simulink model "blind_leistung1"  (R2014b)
settings: Solver=ode8  StartTime=0.0  StopTime=5  FixedStep=1e-5  RelTol=1e-3
undefined symbols (not defined in the file or in its folder): fdesignblkfcn, fir1, gcbh
libraries: dsparch4 x2, dspsigops x1

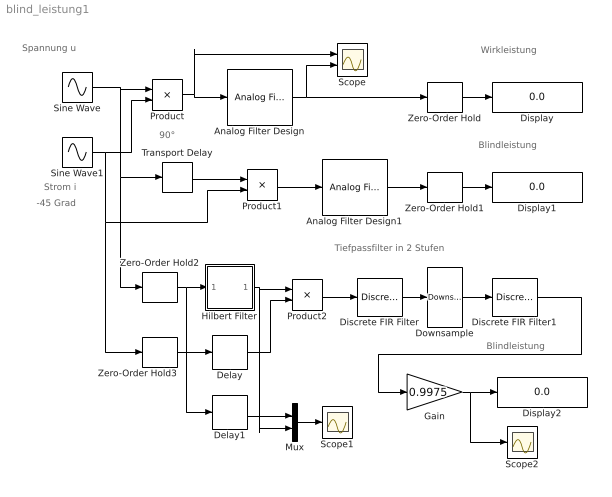
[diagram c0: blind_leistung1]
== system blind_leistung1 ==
  note: Tiefpassfilter in 2 Stufen
  note: Blindleistung
  note: Blindleistung
  note: Wirkleistung
  note: 90°
  note: -45 Grad
  note: Strom i
  note: Spannung u
  Analog Filter Design : dsparch4/Analog Filter Design  method=Butterworth  filttype=Lowpass  N=8  Wlo=2*pi*10  Whi=80  Rp=2  Rs=40
  Analog Filter Design1 : dsparch4/Analog Filter Design  method=Butterworth  filttype=Lowpass  N=8  Wlo=2*pi*10  Whi=80  Rp=2  Rs=40
  Delay : Delay  DelayLength=32
  Delay1 : Delay  DelayLength=32
  Discrete FIR Filter : DiscreteFir  Coefficients=fir1(128, 50*2/1000)
  Discrete FIR Filter1 : DiscreteFir  Coefficients=fir1(128, 10*2/200)
  Display : Display
  Display1 : Display
  Display2 : Display
  Downsample : dspsigops/Downsample  N=5  phase=0  RateOptions=Allow multirate processing  smode=Allow multirate  fmode=Maintain input frame size  ic=0
  Gain : Gain  Gain=0.9975
  Hilbert Filter : Subsystem  DialogController=fdesignblkfcn  InitFcn=fdesignblkfcn(gcbh, {'InitFcn'});
  Mux : Mux  Inputs=2
  Product : Product
  Product1 : Product
  Product2 : Product
  Scope : Scope  NumInputPorts=2
  Scope1 : Scope
  Scope2 : Scope
  Sine Wave : Sin  Amplitude=220  Frequency=2*pi*50  SampleTime=0
  Sine Wave1 : Sin  Amplitude=10.52  Frequency=2*pi*50  Phase=-45*pi/180  SampleTime=0
  Transport Delay : TransportDelay  DelayTime=1/200
  Zero-Order Hold{,1..3} (4 alike) : ZeroOrderHold  SampleTime=1/1000
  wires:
  Sine Wave/1 -> Zero-Order Hold2/1, Transport Delay/1, Product/1
  Sine Wave1/1 -> Zero-Order Hold3/1, Product1/2, Product/2
  Product/1 -> Scope/1, Analog Filter Design/1
  Analog Filter Design/1 -> Scope/2, Zero-Order Hold/1
  Zero-Order Hold/1 -> Display/1
  Transport Delay/1 -> Product1/1
  Product1/1 -> Analog Filter Design1/1
  Zero-Order Hold1/1 -> Display1/1
  Analog Filter Design1/1 -> Zero-Order Hold1/1
  Zero-Order Hold2/1 -> Delay1/1, Hilbert Filter/1(In)
  Zero-Order Hold3/1 -> Delay/1
  Hilbert Filter/1(Out) -> Mux/2, Product2/1
  Delay/1 -> Product2/2
  Discrete FIR Filter/1 -> Downsample/1
  Downsample/1 -> Discrete FIR Filter1/1
  Gain/1 -> Scope2/1, Display2/1
  Discrete FIR Filter1/1 -> Gain/1
  Mux/1 -> Scope1/1
  Delay1/1 -> Mux/1
  Product2/1 -> Discrete FIR Filter/1

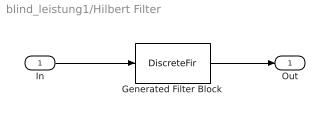
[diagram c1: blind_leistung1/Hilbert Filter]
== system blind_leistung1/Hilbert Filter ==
  In : Inport
  Generated Filter Block : DiscreteFir  Tag=BlockMethodSubSystem  Coefficients=[9.88658825704986609e-06 -0.002227584536743819 -2.97041880887335789e-07 -0.00253443852532551223 3.1215106945712904e-06 -0.00391748816900691285 3.49128676163899538e-06 -0.00575534109882602785 4.57452034469855664e-06 -0.00814133649362377108 5.16425058718461533e-06 -0.0111912068195077624 4.30131386161312988e-06 -0.0150623213220996768 4.89965903312141859e-06 -0.0199570171297331345 4.81145735332042261e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
  Out : Outport
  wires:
  Generated Filter Block/1 -> Out/1
  In/1 -> Generated Filter Block/1
